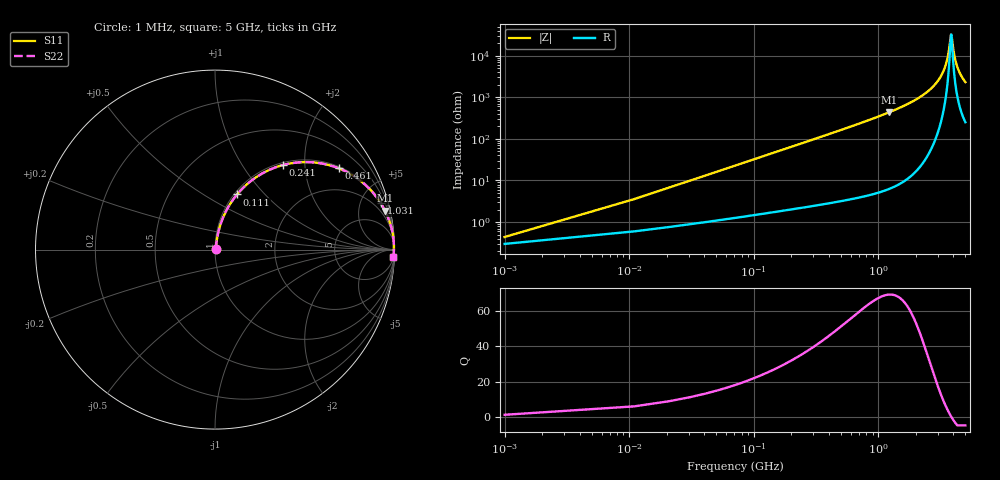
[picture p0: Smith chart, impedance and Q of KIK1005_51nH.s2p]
!version-3
!date-01.2023
!Series
# MHz S RI R 50
!Freq ReS11 ImS11 ReS21 ImS21 ReS12 ImS12 ReS22 ImS22
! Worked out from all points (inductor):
!   501 points, 1 MHz to 5 GHz, reference 50 ohm
!   read as one part in series: L = 51 nH near 21 MHz
!   highest Q = 69.6 at 1.221 GHz (marker M1), where L = 56.7 nH
!   self-resonance near 3.841 GHz
!   S11 on the Smith chart (normalised r, x): 1 MHz: 1.01, +0.01; 111 MHz: 1.03, +0.71; 241 MHz: 1.04, +1.55; 461 MHz: 1.06, +3.00; 1.031 GHz: 1.10, +7.12; 5 GHz: 6, -46
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1  0.00299 0.00319  0.997 -0.00319  0.997 -0.00319  0.00299 0.00319
31  0.0183 0.0967  0.9817 -0.0967  0.9817 -0.0967  0.0183 0.0967
41  0.0264 0.1267  0.9736 -0.1267  0.9736 -0.1267  0.0264 0.1267
71  0.0599 0.2113  0.9401 -0.2113  0.9401 -0.2113  0.0599 0.2113
111  0.1229 0.3075  0.8771 -0.3075  0.8771 -0.3075  0.1229 0.3075
171  0.2393 0.41  0.7607 -0.41  0.7607 -0.41  0.2393 0.41
241  0.3789 0.4712  0.6211 -0.4712  0.6211 -0.4712  0.3789 0.4712
461  0.6885 0.4531  0.3115 -0.4531  0.3115 -0.4531  0.6885 0.4531
841  0.8853 0.311  0.1147 -0.311  0.1147 -0.311  0.8853 0.311
1031  0.9236 0.2584  0.0764 -0.2584  0.0764 -0.2584  0.9236 0.2584
1221  0.947 0.2169  0.053 -0.2169  0.053 -0.2169  0.947 0.2169
1671  0.9754 0.1474  0.0246 -0.1474  0.0246 -0.1474  0.9754 0.1474
2501  0.9928 0.0713  0.00722 -0.0713  0.00722 -0.0713  0.9928 0.0713
2991  0.996 0.041  0.004 -0.041  0.004 -0.041  0.996 0.041
3341  0.9969 0.0228  0.0031 -0.0228  0.0031 -0.0228  0.9969 0.0228
3611  0.9971 0.0102  0.00294 -0.0102  0.00294 -0.0102  0.9971 0.0102
3841  0.9969 0.000264  0.00308 -0.000264  0.00308 -0.000264  0.9969 0.000264
3881  0.9969 -0.0014  0.00312 0.0014  0.00312 0.0014  0.9969 -0.0014
4041  0.9966 -0.00791  0.00337 0.00791  0.00337 0.00791  0.9966 -0.00791
4171  0.9964 -0.013  0.00364 0.013  0.00364 0.013  0.9964 -0.013
4501  0.9954 -0.0253  0.00455 0.0253  0.00455 0.0253  0.9954 -0.0253
5000  0.9935 -0.0425  0.00648 0.0425  0.00648 0.0425  0.9935 -0.0425
